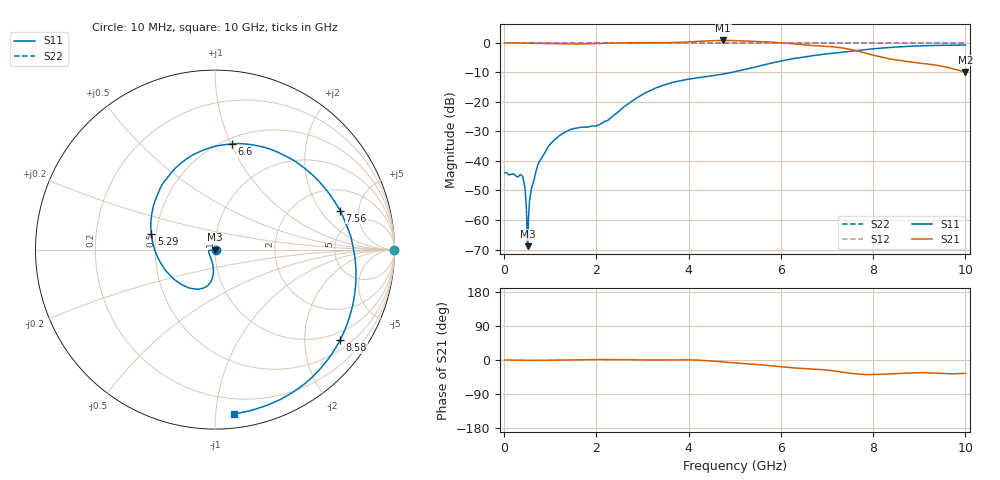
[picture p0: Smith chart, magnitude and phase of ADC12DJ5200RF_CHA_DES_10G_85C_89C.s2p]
! Texas Instruments, Inc.
! ADC12DJ5200RF - CH A S-Parameters (DES Mode, Fs = 10 GSPS, 85 degC case, 89 degC juntion)
! Port 1 represents the 100-ohm differenal input, Port 2 the digital output
! freq  dbS11  angS11  dbS21 angS21 dbS12 angS12 dbS22 angS22
# HZ S DB R 100
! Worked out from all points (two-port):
!   1000 points, 10 MHz to 10 GHz, reference 100 ohm
!   highest |S21| = 0.84 dB at 4.75 GHz (marker M1); lowest = -9.9 dB at 10 GHz (marker M2)
!   |S21| within 3 dB of the highest: start of sweep to 7.496 GHz
!   lowest |S11| = -68.9 dB at 510 MHz (marker M3), VSWR 1.00, Z = 100 - j0.0713 ohm
!   |S11| at or under -10 dB: start of sweep to 4.932 GHz
!   |S22| runs from 0.0 to 0.0 dB; largest |S21 - S12| = 0.76
!   S11 on the Smith chart (normalised r, x): 10 MHz: 1.01, -0.00; 5.29 GHz: 0.47, +0.10; 6.6 GHz: 0.55, +1.01; 7.56 GHz: 3.35, +3.13; 8.58 GHz: 0.75, -2.91; 10 GHz: 0.09, -1.12
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1e7  -43.98 -7.6  0.00 -0.0  0.00 0.0  0.00 0.0
3.8e8  -44.92 -10.5  -0.03 -0.8  0.00 0.0  0.00 0.0
4.3e8  -47.24 -0.5  -0.04 -0.9  0.00 0.0  0.00 0.0
4.7e8  -52.81 6.8  -0.06 -0.9  0.00 0.0  0.00 0.0
5.1e8  -68.87 -81.6  -0.06 -0.9  0.00 0.0  0.00 0.0
6e8  -48.82 -136.8  -0.09 -1.0  0.00 0.0  0.00 0.0
7.1e8  -42.37 -157.4  -0.13 -1.0  0.00 0.0  0.00 0.0
9.4e8  -35.52 -169.1  -0.18 -0.9  0.00 0.0  0.00 0.0
1.26e9  -30.80 -171.7  -0.28 -0.6  0.00 0.0  0.00 0.0
1.68e9  -28.56 -163.4  -0.32 0.6  0.00 0.0  0.00 0.0
2.24e9  -26.25 -119.8  -0.09 1.0  0.00 0.0  0.00 0.0
3.34e9  -14.98 -96.9  0.08 0.1  0.00 0.0  0.00 0.0
4.75e9  -10.53 -156.4  0.84 -5.2  0.00 0.0  0.00 0.0
5.01e9  -9.74 -174.4  0.79 -7.9  0.00 0.0  0.00 0.0
5.29e9  -8.74 165.9  0.62 -10.3  0.00 0.0  0.00 0.0
5.9e9  -6.49 126.2  0.16 -16.6  0.00 0.0  0.00 0.0
6.6e9  -4.49 81.1  -0.75 -23.3  0.00 0.0  0.00 0.0
6.67e9  -4.33 76.5  -0.85 -23.8  0.00 0.0  0.00 0.0
7.56e9  -2.73 17.4  -2.37 -35.8  0.00 0.0  0.00 0.0
8.34e9  -1.56 -25.8  -5.35 -36.9  0.00 0.0  0.00 0.0
8.58e9  -1.31 -35.9  -5.91 -35.5  0.00 0.0  0.00 0.0
1e10  -0.71 -83.2  -9.86 -35.2  0.00 0.0  0.00 0.0
